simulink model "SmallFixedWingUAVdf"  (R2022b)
settings: Solver=ode4  StartTime=0.01  StopTime=50  FixedStep=0.001  RelTol=1e-3  EnableMultiTasking=on
PreLoadFcn:
  | asbswarm_vehicledata; % load in workspace variables
PostLoadFcn:
  | open_system([gcs,'/MATLAB Animation Display/MATLAB',10,'Animation']);
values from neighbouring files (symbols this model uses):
  uav = struct    [InitDatactrldf.m]    (also in InitDatactrl.m)
undefined symbols (not defined in the file or in its folder): Busy, Wait
libraries: aerolibptmass x1, aerolibanimutils x1

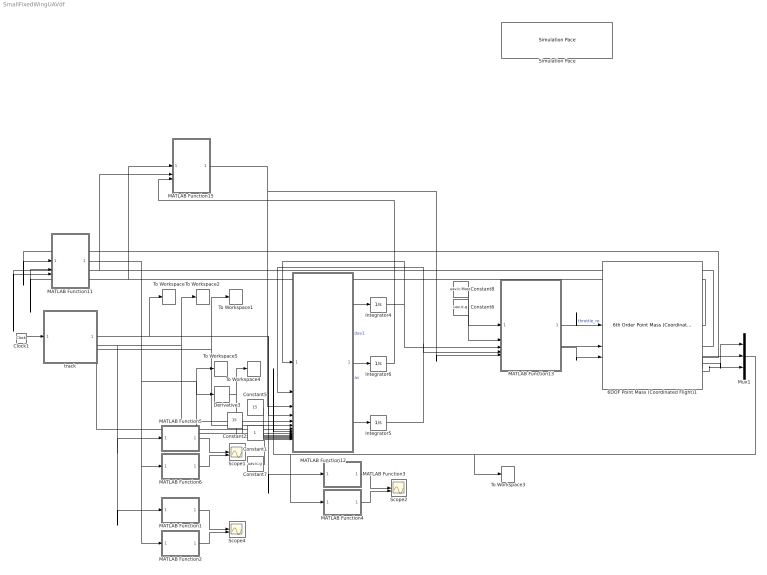
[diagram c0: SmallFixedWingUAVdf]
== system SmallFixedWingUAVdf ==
  6DOF Point Mass (Coordinated Flight)1 : aerolibptmass/6th Order Point Mass (Coordinated Flight)  units=Metric (MKS)  gamma0=uav.ic.Gam  chi0=uav.ic.Chi  V0=uav.ic.V  x0=uav.ic.East  y0=uav.ic.North  h0=uav.ic.Up  mass0=uav.ic.Mass
  Clock1 : Clock
  Constant1 : Constant
  Constant2 : Constant  Value=15
  Constant5 : Constant  Value=15
  Constant6 : Constant  Value=uav.ic.g
  Constant7 : Constant  Value=uav.ic.g
  Constant8 : Constant  Value=uav.ic.Mass
  Derivative3 : Derivative
  Integrator4 : Integrator
  Integrator5 : Integrator
  Integrator6 : Integrator
  MATLAB Function1 : MATLAB Function  TreatAsAtomicUnit=on
  MATLAB Function11 : MATLAB Function  TreatAsAtomicUnit=on
  MATLAB Function12 : MATLAB Function  TreatAsAtomicUnit=on
  MATLAB Function13 : MATLAB Function  TreatAsAtomicUnit=on
  MATLAB Function15 : MATLAB Function  TreatAsAtomicUnit=on
  MATLAB Function2 : MATLAB Function  TreatAsAtomicUnit=on
  MATLAB Function3 : MATLAB Function  TreatAsAtomicUnit=on
  MATLAB Function4 : MATLAB Function  TreatAsAtomicUnit=on
  MATLAB Function5 : MATLAB Function  TreatAsAtomicUnit=on
  MATLAB Function6 : MATLAB Function  TreatAsAtomicUnit=on
  Mux1 : Mux  Inputs=3
  Scope1 : Scope  NumInputPorts=2
  Scope2 : Scope  NumInputPorts=2
  Scope4 : Scope  NumInputPorts=2
  Simulation Pace : aerolibanimutils/Simulation Pace  SimulationPace=1  SleepMode=Busy-Wait  OutputPaceError=off  SampleTime=-1
  To Workspace : ToWorkspace  VariableName=Xd  SampleTime=0.1
  To Workspace1 : ToWorkspace  VariableName=Ad  SampleTime=0.1
  To Workspace2 : ToWorkspace  VariableName=Vd  SampleTime=0.1
  To Workspace3 : ToWorkspace  VariableName=X  SampleTime=0.1
  To Workspace4 : ToWorkspace  VariableName=A  SampleTime=0.1
  To Workspace5 : ToWorkspace  VariableName=V  SampleTime=0.1
  track : MATLAB Function  TreatAsAtomicUnit=on
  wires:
  Constant5/1 -> MATLAB Function12/11(k1)
  Constant6/1 -> MATLAB Function13/2(g)
  Integrator5/1 -> MATLAB Function13/4(av3), MATLAB Function12/2(av3)
  MATLAB Function12/1(dav1) -> Integrator4/1  "dav1"
  Integrator4/1 -> MATLAB Function12/1(av1), MATLAB Function13/3(av1)
  track/3(Ad) -> To Workspace1/1, MATLAB Function12/6(ddxd)
  Clock1/1 -> track/1(t)
  track/2(Vd) -> MATLAB Function1/1(u), MATLAB Function5/1(u), To Workspace2/1, MATLAB Function12/5(dxd)
  Derivative3/1 -> To Workspace4/1, MATLAB Function12/10(ddx)
  MATLAB Function12/3(dav3) -> Integrator5/1
  Constant7/1 -> MATLAB Function12/14(g)
  track/4(Jd) -> MATLAB Function12/7(dddxd)
  MATLAB Function13/2(Fy) -> 6DOF Point Mass (Coordinated Flight)1/2
  MATLAB Function13/1(Fx) -> 6DOF Point Mass (Coordinated Flight)1/1  "throttle_re"
  MATLAB Function13/3(Fz) -> 6DOF Point Mass (Coordinated Flight)1/3
  Constant8/1 -> MATLAB Function13/1(m)
  6DOF Point Mass (Coordinated Flight)1/3 -> MATLAB Function11/1(Velocity)
  6DOF Point Mass (Coordinated Flight)1/1 -> MATLAB Function15/1(gamma), MATLAB Function11/2(gamma)
  6DOF Point Mass (Coordinated Flight)1/2 -> MATLAB Function15/2(chi), MATLAB Function11/3(chi)
  MATLAB Function11/1(dx) -> To Workspace5/1, MATLAB Function12/9(dx), Derivative3/1, MATLAB Function6/1(u), MATLAB Function2/1(u)
  MATLAB Function12/2(w1) -> Integrator6/1  "av"
  Integrator6/1 -> MATLAB Function15/3(mu)
  MATLAB Function15/1(R) -> MATLAB Function13/5(R), MATLAB Function12/3(R)
  MATLAB Function5/1(y) -> Scope1/1
  MATLAB Function6/1(y) -> Scope1/2
  MATLAB Function1/1(y) -> Scope4/1
  MATLAB Function2/1(y) -> Scope4/2
  6DOF Point Mass (Coordinated Flight)1/5 -> Mux1/2
  6DOF Point Mass (Coordinated Flight)1/6 -> Mux1/3
  track/1(Xd) -> To Workspace/1, MATLAB Function3/1(u), MATLAB Function12/4(xd)
  6DOF Point Mass (Coordinated Flight)1/4 -> Mux1/1
  Mux1/1 -> To Workspace3/1, MATLAB Function12/8(x), MATLAB Function4/1(u)
  MATLAB Function4/1(y) -> Scope2/2
  MATLAB Function3/1(y) -> Scope2/1
  Constant1/1 -> MATLAB Function12/13(k3)
  Constant2/1 -> MATLAB Function12/12(k2)

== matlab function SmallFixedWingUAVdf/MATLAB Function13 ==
function [Fx,Fy,Fz] = fcn(m,g,av1,av3,R)
N=3;
Fxyz=zeros(N,1);

av = [av1;0;av3];
a = [0;0;-g]+R*av;
Fxyz = R'*(m*a);
Fx=Fxyz(1);
Fy=Fxyz(2);
Fz=Fxyz(3);

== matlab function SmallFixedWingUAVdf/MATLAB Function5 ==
function y = fcn(u)

y = u(1);

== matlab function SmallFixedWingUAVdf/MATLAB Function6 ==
function y = fcn(u)

y = u(1);

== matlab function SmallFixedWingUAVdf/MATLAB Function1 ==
function y = fcn(u)

y = u(2);

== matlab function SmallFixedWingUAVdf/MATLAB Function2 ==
function y = fcn(u)

y = u(2);

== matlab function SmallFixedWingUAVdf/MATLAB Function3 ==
function y = fcn(u)

y = u(2);

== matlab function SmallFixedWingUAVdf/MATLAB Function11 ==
function dx = fcn(Velocity,gamma,chi)
 
%     dx(i,:)=[Velocity(i)*cos(gamma(i))*cos(chi(i)),Velocity(i)*sin(gamma(i))*cos(chi(i)),Velocity(i)*sin(gamma(i))];
    dx=[Velocity*cos(chi)*cos(gamma),Velocity*sin(chi)*cos(gamma),Velocity*sin(gamma)]';

end

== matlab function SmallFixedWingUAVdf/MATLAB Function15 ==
function R = fcn(gamma,chi,mu)
    roll = mu;
    pitch = gamma;
    yaw = chi;

    R = ROTZ(yaw)*ROTX(roll)*ROTY(pitch);
end

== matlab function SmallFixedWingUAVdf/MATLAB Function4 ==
function y = fcn(u)

y = u(2);

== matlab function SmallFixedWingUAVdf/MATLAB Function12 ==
function [dav1,w1,dav3] = DF(av1,av3,R,xd,dxd,ddxd,dddxd,x,dx,ddx,k1,k2,k3,g)
    dav1=zeros(1,1);
    w1=zeros(1,1);
    dav3=zeros(1,1);
    
    V = norm(dx,2);
    gv = R'*[0;0;-g];
    w2=-(av3+gv(3))/V;
    w3=gv(2)/V;

    u = dddxd + k1*(ddxd-ddx) + k2*(dxd-dx)+ k3*(xd-x);

    a = [-w2*av3;w3*av1/av3;w2*av1];
    B = [1,0,0;0,-1/av3,0;0,0,1];
    out = a + B*R'*u;

    dav1=out(1); w1=out(2); dav3=out(3);

    if isnan(dav1)
        dav1=0;
    end
    if isnan(w1)
        w1=0;
    end
    if isnan(dav3)
        dav3=0;
    end

end

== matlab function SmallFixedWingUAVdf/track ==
function [Xd,Vd,Ad,Jd] = fcn(t)
Xd=[4*t-cos(t),-0.5*cos(2*t),10+sin(t)]';
Vd=[4+sin(t),sin(2*t),cos(t)]';
Ad=[cos(t),2*cos(2*t),-sin(t)]';
Jd=[-sin(t),-4*sin(2*t),-cos(t)]';
end
